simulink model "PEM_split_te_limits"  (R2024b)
settings: Solver=VariableStepAuto  StartTime=0.0  StopTime=t_end  MaxStep=10  RelTol=1e-3
model workspace (MAT data in the model file):
  F_farad = 96485.332
  HHV_H2 = 285.8
  M_H2 = 2.0159
  R = 8.314462
  T_std = 298.15
  Ta = 288.15
  V_std = 1.23
  V_th = 1.48
  cp_H2_coeff = [29.11 -0.00192 4e-06 -8.7e-10]
  cp_O2_coeff = [25.48 0.0152 -7.16e-06 1.31e-09]
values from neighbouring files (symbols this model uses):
  A_new = 5000    [ely_therm_sub_model.m]    (also in run_nl_PEM_split_thermal_elchem.m)
  N_new = 75    [ely_therm_sub_model.m]    (also in run_nl_PEM_split_thermal_elchem.m)
  p_an = 29    [run_nl_PEM_split_thermal_elchem.m]
  p_cat = 30    [run_nl_PEM_split_thermal_elchem.m]

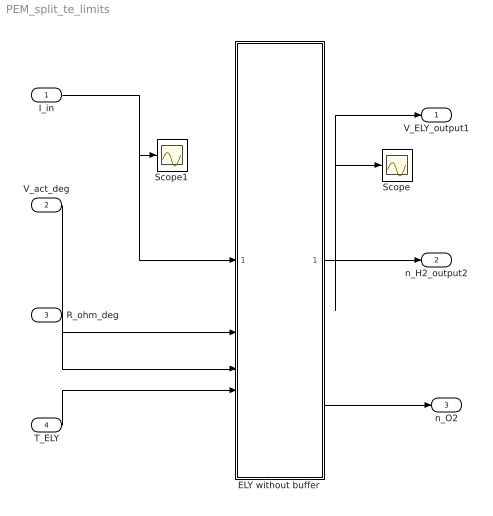
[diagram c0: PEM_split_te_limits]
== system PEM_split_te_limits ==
  I_in : Inport
  V_act_deg : Inport  Port=2
  R_ohm_deg : Inport  Port=3
  T_ELY : Inport  Port=4
  ELY without buffer : Subsystem
  Scope : Scope
  Scope1 : Scope
  V_ELY_output1 : Outport
  n_H2_output2 : Outport  Port=2
  n_O2 : Outport  Port=3
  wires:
  R_ohm_deg/1 -> ELY without buffer/3(R_ohm_deg)
  V_act_deg/1 -> ELY without buffer/2(V_act_deg)
  I_in/1 -> Scope1/1, ELY without buffer/1(I_in)
  ELY without buffer/1(V_ELY) -> V_ELY_output1/1, Scope/1
  T_ELY/1 -> ELY without buffer/4(T_ELY)
  ELY without buffer/3(n_O2) -> n_O2/1
  ELY without buffer/2(n_H2) -> n_H2_output2/1

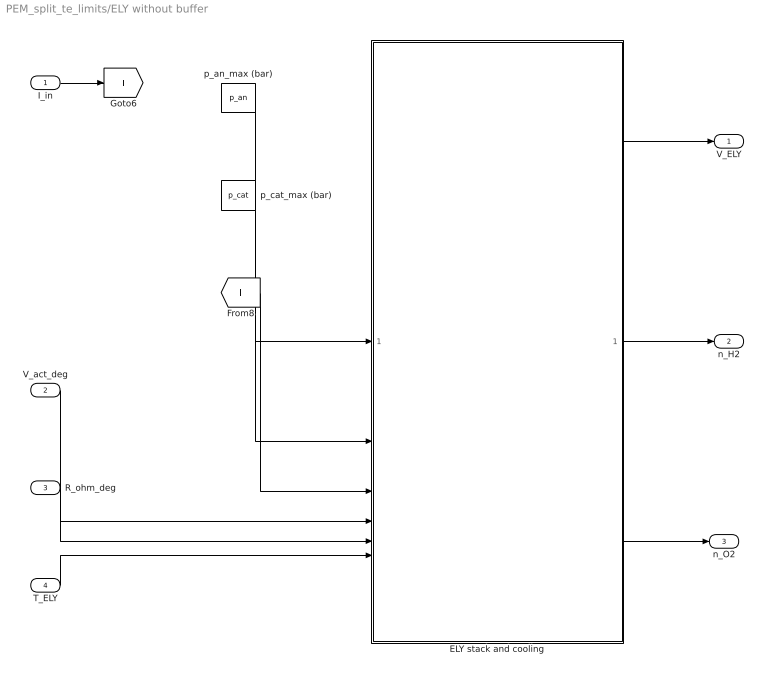
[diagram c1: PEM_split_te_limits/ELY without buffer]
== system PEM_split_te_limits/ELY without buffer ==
  I_in : Inport
  V_act_deg : Inport  Port=2
  R_ohm_deg : Inport  Port=3
  T_ELY : Inport  Port=4
  ELY stack and cooling : Subsystem
      mask init:
      | % for 400 A
      | %x0Temp1=333.1500;
      | %x0Temp2=3.329024438021895e+02;
      | %x0Qpi=5.618311056096404e+03;
      | %x0V_act=19.360033620504169;
      | 
      | %P_Q=-1662.44867463832; I_Q=-25.4752882159372;
  p_an_max (bar) : Constant  Value=p_an
  p_cat_max (bar) : Constant  Value=p_cat
  V_ELY : Outport
  n_H2 : Outport  Port=2
  n_O2 : Outport  Port=3
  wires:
  V_act_deg/1 -> ELY stack and cooling/4(V_act_deg)
  I_in/1 -> [I]
  R_ohm_deg/1 -> ELY stack and cooling/5(R_ohm_deg)
  p_an_max (bar)/1 -> ELY stack and cooling/1(p_an)
  ELY stack and cooling/1(V_ELY (V)) -> V_ELY/1
  p_cat_max (bar)/1 -> ELY stack and cooling/2(p_cat)
  [I] -> ELY stack and cooling/3(I)
  ELY stack and cooling/2(n_H2) -> n_H2/1
  ELY stack and cooling/3(n_O2) -> n_O2/1
  T_ELY/1 -> ELY stack and cooling/6(T_ELY)

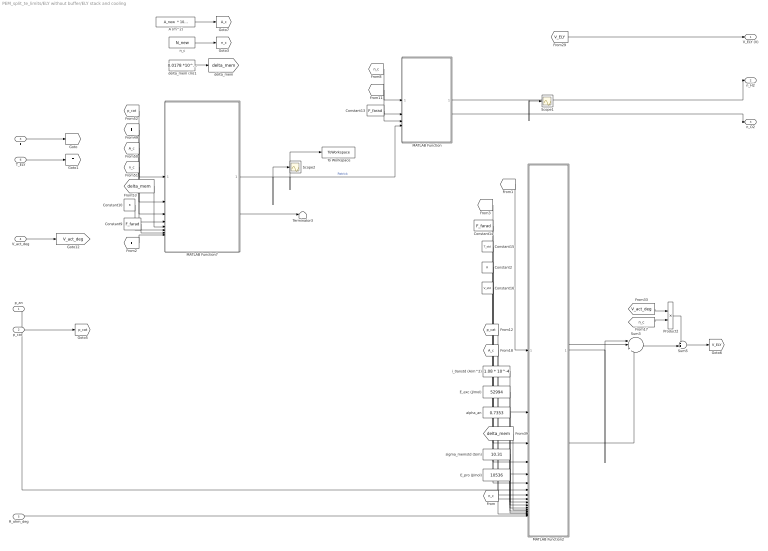
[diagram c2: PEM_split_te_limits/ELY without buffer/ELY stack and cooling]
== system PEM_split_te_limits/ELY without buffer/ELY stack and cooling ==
  p_an : Inport
  p_cat : Inport  Port=2
  I : Inport  Port=3
  V_act_deg : Inport  Port=4
  R_ohm_deg : Inport  Port=5
  T_ELY : Inport  Port=6
  A (m^2) : Constant  Value="A_new  * 10^-4"
  Constant10 : Constant  Value=R
  Constant13 : Constant  Value=F_farad
  Constant14 : Constant  Value=F_farad
  Constant15 : Constant  Value=T_std
  Constant16 : Constant  Value=V_std
  Constant2 : Constant  Value=R
  Constant9 : Constant  Value=F_farad
  E_exc (J/mol) : Constant  Value=52994
  E_pro (J/mol) : Constant  Value=10536
  MATLAB Function : MATLAB Function  TreatAsAtomicUnit=on
  MATLAB Function2 : MATLAB Function  TreatAsAtomicUnit=on
  MATLAB Function7 : MATLAB Function  TreatAsAtomicUnit=on
  Product2 : Product
  Scope1 : Scope
  Scope2 : Scope
  Sum3 : Sum  Inputs=|+++
  Sum5 : Sum  Inputs=++|
  Terminator3 : Terminator
  To Workspace : ToWorkspace  VariableName=eta_H2  SaveFormat=Timeseries  SampleTime=-1
  alpha_an : Constant  Value=0.7353
  delta_mem (m)1 : Constant  Value=0.0178 *10^-2
  i_0anstd (A/m^2) : Constant  Value=1.08 * 10^-4
  n_c : Constant  Value=N_new
  sigma_memstd (S/m) : Constant  Value=10.31
  V_ELY (V) : Outport
  n_H2 : Outport  Port=2
  n_O2 : Outport  Port=3
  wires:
  p_an/1 -> MATLAB Function2/7(p_an)
  p_cat/1 -> [p_cat]
  Constant14/1 -> MATLAB Function2/3(F)
  E_pro (J/mol)/1 -> MATLAB Function2/15(E_pro)
  n_c/1 -> [n_c]
  i_0anstd (A/m^2)/1 -> MATLAB Function2/10(i_0anstd)
  alpha_an/1 -> MATLAB Function2/12(alpha_an)
  E_exc (J/mol)/1 -> MATLAB Function2/11(E_exc)
  [I] -> MATLAB Function2/1(I)
  [delta_mem] -> MATLAB Function2/13(delta_mem)
  Constant15/1 -> MATLAB Function2/4(T_std)
  Constant13/1 -> MATLAB Function/3(F)
  sigma_memstd (S/m)/1 -> MATLAB Function2/14(sigma_memstd)
  [A_c] -> MATLAB Function2/9(A)
  MATLAB Function/2(n_O2) -> n_O2/1
  [n_c] -> MATLAB Function/1(n_c)
  [I] -> MATLAB Function/2(I)
  I/1 -> [I]
  MATLAB Function/1(n_H2) -> Scope1/1, n_H2/1
  MATLAB Function2/3(V_act) -> Sum3/3
  MATLAB Function2/1(V_ocv) -> Sum3/1
  MATLAB Function2/2(V_ohm) -> Sum3/2
  [n_c] -> MATLAB Function2/16(n_c)
  [V_ELY] -> V_ELY (V)/1
  A (m^2)/1 -> [A_c]
  Constant2/1 -> MATLAB Function2/5(R)
  Constant16/1 -> MATLAB Function2/6(V_std)
  R_ohm_deg/1 -> MATLAB Function2/17(R_ohm_deg)
  [p_cat] -> MATLAB Function2/8(p_cat)
  delta_mem (m)1/1 -> [delta_mem]
  V_act_deg/1 -> [V_act_deg]
  [V_act_deg] -> Product2/1
  Sum5/1 -> [V_ELY]
  Sum3/1 -> Sum5/2
  [n_c] -> Product2/2
  Product2/1 -> Sum5/1
  [p_cat] -> MATLAB Function7/1(p_h2)
  [delta_mem] -> MATLAB Function7/5(delta_mem)
  [A_c] -> MATLAB Function7/3(A_cell)
  MATLAB Function7/1(eta_fara_h2) -> Scope2/1, To Workspace/1, MATLAB Function/4(nF)  "Patrick"
  [I] -> MATLAB Function7/2(I)
  [n_c] -> MATLAB Function7/4(n_cell)
  MATLAB Function7/2(h2_o2) -> Terminator3/1
  Constant9/1 -> MATLAB Function7/7(F)
  Constant10/1 -> MATLAB Function7/6(R)
  T_ELY/1 -> [T]
  [T] -> MATLAB Function7/8(T)
  [T] -> MATLAB Function2/2(T)

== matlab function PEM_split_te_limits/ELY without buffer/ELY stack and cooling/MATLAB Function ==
function [n_H2,n_O2] = productionH2O2(n_c,I,F,nF)

%Hydrogen and oxygen prodcution of electrolyzer

%(as long not other noted, inputs and outputs are scalar values)
%inputs:
% n_c       - number of cells                   - /
% I         - DC current                        - A
% F         - Faraday's constant                - C/mol
% nF        - Faraday's efficiency              - /

%outputs:
% n_H2      - produced H2 stream                - mol/s
% n_O2      - produced O2 stream                - mol/s

%--------------------------------------------------------------------------


n_H2 = ((n_c*I)/(2*F))*nF;

n_O2 = n_H2/2;

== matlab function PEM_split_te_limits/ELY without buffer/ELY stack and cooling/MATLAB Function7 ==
function [eta_fara_h2, h2_o2] = faraday_efficiency_Patrick(p_h2,I, A_cell,n_cell,delta_mem,R,F,T)
%Crossover Model von Patrick Trinke
% inputs:
% p_h2   - hydrogen pressure        - in bar 
% I      - electrolyzer current     - in A
% A_cell - cross section of the studied PEM electrolyzer - in m^2
% n_cell - number of cells          - /
% delta_mem - membrane thickness    - m
% R - ideal gas constant            - J/(mol K)
% F - faraday constant              - As/mol 
% T - Temperature                   - K
% outputs: 
% eta_fara_h2 - faraday efficiency  - in /
% h2_o2  - H2 in O2                 - in in vol.%
%


%% Eingangparameter
% Kathodendruck
p_h2 = p_h2 * 1e5; % Pa


%% Parameter
% Diffusionskoeff:
% Dummy: D_h2 = 5e-9; % m²/s
% Dis Patrick, S. 110 Tab. A2, Eq. (A.6)
%Mail: 08.09.2023 In meiner Diss habe ich die Werte D_h0 und Do0 falsch mit e-7 angegeben. Richtig ist e-6 also sind die Diffusionskoeffzienten eine Zehnerpotenz größer.
%old: D_dsg_h2_T_0 = 4.9e-7; %m^2/s  
%new:
D_dsg_h2_T_0 = 4.9e-6; %m^2/s  
E_h2 = 16.51e3; %J/mol
D_dsg_h2_T = D_dsg_h2_T_0 * exp(-E_h2/(R*T));
% Dis Patrick, S. 61 Eq. (6.9)
eps_ion = 1; % Ionomer fraction in the membrane Tab. 6.1 
eps_H2O = 0.42; %Tab. 4.2 = 0.37 / Tab. 5.1 = 0.42 / εH2O the water fraction within the ionomer,
tau_ion = 1.5; %Tab. 4.2 same in Tab. 1.5 / tortuosity of the ionomer channels
D_eff_dsg_h2 = ((eps_ion*eps_H2O)/tau_ion)*D_dsg_h2_T;

%D_eff_dsg_h2 = 5e-9; % m²/s

% Löslichkeitskonstante
%Dummy value: S_h2 = 7e-6; % mol/m³/Pa
% Dis Patrick, S. 110 Tab. A2, Eq. (A.7)
A_h2 = -48.1611;
B_h2 = 5528.45;
C_h2 = 16.8893;
S_h2 = 0.55*exp(A_h2+B_h2/T+C_h2*log(T/100)); %T in K / result in mol/m³/Pa

% Faradaykonstante
%F = 96485; % As/mol 

% Mass transfer coefficient
% Dis Patrick, S. 38 Fig. 4.5 / material dependent / chosen value
k_l = 3e-2; % m/s


%% Geometrische Werte
% Membrandicke
%delta_mem = 125e-6; % m
% Zellfläche (Grundfläche)
%A_cell = 0.5; % m²
% Zellanzahl
%n_cell = 50; % #

% Stackfläche 
A_stack = A_cell * n_cell; % m²


%% Berechnungen:

% produzierte Gasströme
o2_evo = I/4/F * n_cell; % mol/s
h2_evo = I/2/F * n_cell; % mol/s

% Übersättigte Wasserstoffkonzentration in der Kathode https://www.sciencedirect.com/science/article/abs/pii/S0360319917312971 
c_h2_super = (I/A_cell/2/F + k_l*p_h2*S_h2) / (k_l + D_eff_dsg_h2/delta_mem)  ; % mol/m³

% Crossoverfluss für den gesamten Stack
N_h2_cross_stack = D_eff_dsg_h2 * c_h2_super/delta_mem * A_stack; % mol/s

% H2 in O2
h2_o2 = N_h2_cross_stack / (N_h2_cross_stack + o2_evo) * 100; % in vol.%

% Faraday Wirkungsgrad
eta_fara_h2 = (1 - N_h2_cross_stack / h2_evo ); % in - 


% Notes: D, k_l und delta_mem sind potentielle Parameter die Altern
% könnten. D und S haben Temperaturabhängigkeiten
% Zur Crossover Theorie kannst du dir gerne das Paper angucken: https://www.sciencedirect.com/science/article/abs/pii/S0360319917312971

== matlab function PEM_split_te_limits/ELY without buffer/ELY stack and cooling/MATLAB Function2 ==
  function [V_ocv,V_ohm,V_act] = Electrochem_model(I,T,F,T_std,R,V_std,p_an,p_cat,A,i_0anstd,E_exc,...
    alpha_an,delta_mem,sigma_memstd,E_pro,n_c,R_ohm_deg)
%
%Electrochemical sub-model of electrolyzer for calculation of cell voltage
%
%(as long not other noted, inputs and outputs are scalar values)
%inputs:
% I         - DC current                        - A
% T         - cell temperature                  - K 
% F         - Faraday's constant                - C/mol
% T_std     - standard temperature              - K 
% R         - universal gas constant            - J/(mol K)
% V_std     - standard cell voltage             - V
% p_an      - anodic pressure                   - bar 
% p_cat     - cathodic pressure                 - bar 
% A         - Active catalyst area              - m^2
% i_0anstd  - electrode exchange current density anode standard - A/m^2
% (i_0anstd from Webster et al.)
% E_exc     - activation energy required for the electron transport in
% the anode electrode - J/mol
% alpha_an  - charge transfer coefficient anode - /
% delta_mem - membrane thickness                - m
% sigma_memstd - protonic conductivity          - S/m
% E_pro     - activation energy required for the proton transport in
% the membrane                                  - J/mol
% V_act     - activation overpotential          - V
% n_c       - number of cells                   - - 
%
%outputs:
% I_farad - Faraday current                     - A
% V_ocv - open circuit voltage                  - V
% V_ohm - ohmic voltage                         - V
% dVactdt - change of activation voltage        - V/s
%% ------------------------------------------------------------------------

i = I/A;                    % in A/m^2

p_an = p_an/1.01325;        %bar in atm
p_cat = p_cat/1.01325;      %bar in atm

%% ------------ open-circuit voltage --------------------------------------

V_rev = V_std - 0.0009*(T-T_std);

% Esp. Eq. (5)-(7)
p_H2O = 6.1078*10^-3*exp(17.2694*((T-273.15)/(T-34.85))); %in atm!!!
p_H2 = p_cat - p_H2O; %in atm
p_O2 = p_an - p_H2O; %in atm

%Durckabhängigkeit Ggw.-spannung
V_ocv_cell = V_rev + ((R*T)/(2*F))*(log((p_H2*p_O2^0.5)/p_H2O));
V_ocv = V_ocv_cell * n_c;
%% ------------activation overvoltage -------------------------------------
% Esp. Eq. (11)
i_0an = i_0anstd*exp(-(E_exc/R)*(1/T-1/T_std)); % A/m^2

%activation overpotential 
%Volmer-Butler-Equation (Esp. Eq. (10))
V_act = ((R*T)/(2*alpha_an*F))*asinh(i/(2*i_0an))*n_c;


%% ------------ohmic overvoltage-------------------------------------------
% Esp. Eq. (16)
sigma_mem = sigma_memstd*exp(-(E_pro/R)*(1/T-1/T_std)); % in S/m
% Esp. Eq. (14)
R_mem = delta_mem / sigma_mem; % m/(S/m) = m^2/S = Ohm m^2
%considering degradation
R_mem_tot = R_mem + R_ohm_deg;
% Esp. Eq. (13)
V_ohm = R_mem_tot * i *n_c; %total for whole stack (*n_c) / Ohm m^2 * A/m^2 = V
